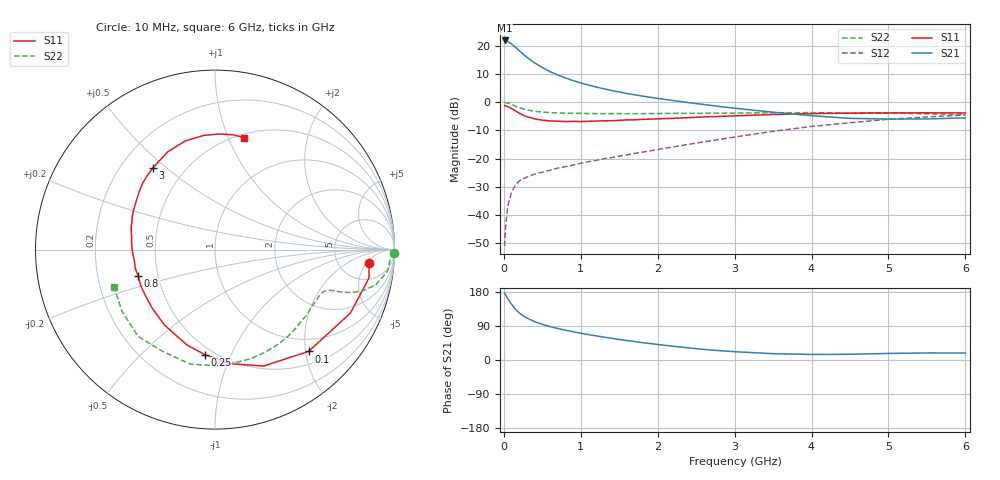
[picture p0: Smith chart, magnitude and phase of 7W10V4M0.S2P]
! Infineon Technologies  Discrete & RF Semiconductors
! BFS17W
! Si NPN RF Bipolar Junction Transistor in SOT323
! VCE = 10 V  IC = 4 mA
! Common Emitter S-Parameters:  August  1999
# GHz  S  MA  R  50
!  f  S11  S21  S12  S22
! GHz  MAG  ANG  MAG  ANG  MAG  ANG  MAG  ANG
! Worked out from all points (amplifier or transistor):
!   36 points, 10 MHz to 6 GHz, reference 50 ohm
!   highest |S21| = 21.9 dB at 10 MHz (marker M1)
!   |S21| within 3 dB of that: start of sweep to 174.9 MHz
!   unconditionally stable (mu >= 1): 666.5 MHz to 2.358 GHz; 5.229 GHz to end of sweep
!   at 250 MHz: K = 0.51, MSG = 22.1 dB, |S12| = -27.2 dB
!   at 1.4 GHz: K = 1.21, MAG = 9.1 dB, |S12| = -19.7 dB
!   at 6 GHz: K = 1.05, MAG = -1.9 dB, |S12| = -4.5 dB
!   S11 on the Smith chart (normalised r, x): 10 MHz: 10, -6; 100 MHz: 0.74, -2.06; 250 MHz: 0.45, -0.80; 800 MHz: 0.39, -0.14; 3 GHz: 0.33, +0.45; 6 GHz: 0.54, +1.14
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0.01  0.8619 -5.0  12.42 176.7  0.0028 85.5  0.9977 -1.0
0.02  0.8724 -10.4  12.42 172.6  0.0055 85.1  0.9779 -2.8
0.05  0.8333 -25.1  11.95 162.1  0.0141 79.1  0.9701 -7.0
0.1  0.7705 -47.4  10.76 147.0  0.0253 67.7  0.9159 -12.5
0.15  0.7031 -67.3  9.44 134.1  0.0339 58.5  0.851 -15.7
0.2  0.6408 -82.7  8.186 124.5  0.0402 55.3  0.7994 -17.4
0.25  0.5874 -95.6  7.109 116.9  0.0437 51.7  0.7578 -18.3
0.3  0.5534 -106.5  6.247 110.7  0.0472 50.5  0.7288 -18.7
0.4  0.5061 -123.7  4.979 101.1  0.053 49.6  0.6894 -19.3
0.5  0.4793 -136.4  4.113 94.0  0.0574 50.3  0.6677 -19.8
0.6  0.4652 -146.3  3.482 88.2  0.0622 51.8  0.6537 -20.7
0.8  0.4526 -161.2  2.695 78.6  0.0721 55.2  0.638 -23.3
0.9  0.4566 -167.0  2.413 74.6  0.0764 56.9  0.6329 -24.6
1.1  0.4585 -177.0  2.011 66.9  0.0881 59.7  0.6288 -28.1
1.3  0.4672 174.7  1.728 60.4  0.099 62.3  0.6254 -32.0
1.6  0.4849 164.5  1.426 51.3  0.1166 65.6  0.6248 -38.1
2.2  0.5172 147.8  1.069 36.3  0.161 70.7  0.6325 -52.0
3  0.5716 127.3  0.782 21.9  0.2409 71.6  0.6395 -72.3
3.5  0.6051 115.8  0.664 16.7  0.3045 69.0  0.6496 -86.4
4.5  0.6394 95.6  0.516 15.1  0.4316 57.6  0.6379 -117.1
5.5  0.6479 81.1  0.504 18.6  0.5481 44.1  0.6217 -146.6
6  0.6442 75.5  0.527 18.5  0.5932 37.4  0.5998 -159.8
